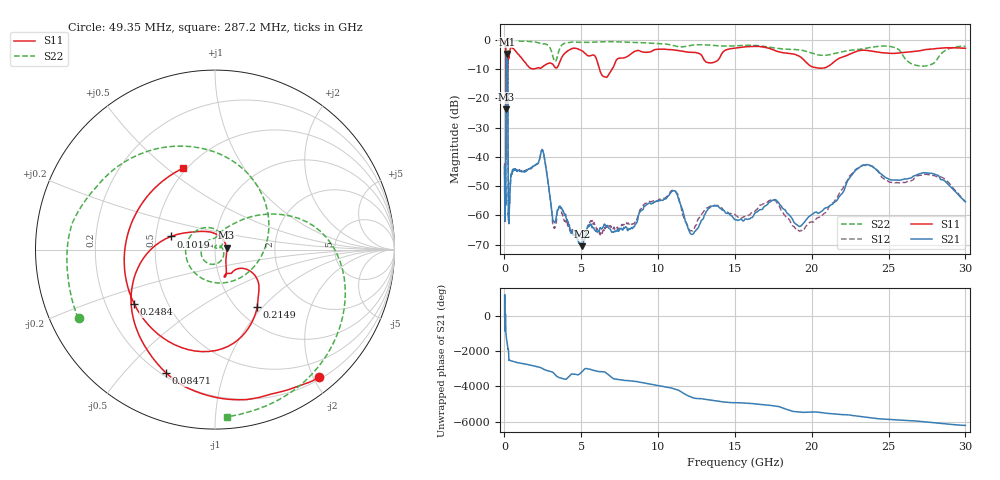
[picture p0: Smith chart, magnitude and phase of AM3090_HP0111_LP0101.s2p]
! Date/Time: Thu, Feb 28, 2019 2:01 PM
! Network Analyzer: Agilent Technologies E8364B Rev: A.07.50.67
! Sweep from 0.010 to 30.000 GHz, 1601 Points, Sweep Type: LOG
! Power Supply: 5.023 V, 0.002 A
# Hz S DB R 50
!freq MagS11 AngS11 MagS21 AngS21 MagS12 AngS12 MagS22 AngS22
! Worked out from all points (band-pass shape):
!   1601 points, 10 MHz to 30 GHz, reference 50 ohm
!   highest |S21| = -4.75 dB at 153.7 MHz (marker M1); lowest = -70.6 dB at 5.077 GHz (marker M2)
!   |S21| within 3 dB of the highest: 113.2 MHz to 202.8 MHz (89.6 MHz wide, 56.7 % of centre)
!   lowest |S11| = -23.7 dB at 109.9 MHz (marker M3), VSWR 1.14, Z = 56.8 + j1.22 ohm
!   |S11| at or under -10 dB: 100.8 MHz to 204 MHz (103.2 MHz wide, 67.7 % of centre); 6.184 GHz to 7.009 GHz (825 MHz wide, 12.5 % of centre)
!   |S22| runs from -40.8 to -0.1 dB; largest |S21 - S12| = 0.013
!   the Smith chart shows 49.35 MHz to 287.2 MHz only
!   S11 on the Smith chart (normalised r, x): 49.35 MHz: 0.23, -2.09; 84.71 MHz: 0.22, -0.66; 101.9 MHz: 0.60, +0.09; 214.9 MHz: 1.23, -0.93; 248.4 MHz: 0.32, -0.27; 287.2 MHz: 0.48, +0.57
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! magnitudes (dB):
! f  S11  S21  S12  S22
! 10 MHz  -0.3  -47.2  -42.2  -0.6
! 38.04 MHz  -0.5  -60.3  -61.3  -1.3
! 49.35 MHz  -0.7  -50.5  -47.1  -1.4
! 84.71 MHz  -2.6  -51.2  -49.8  -5.3
! 101.9 MHz  -11.9  -17.1  -17.1  -15.1
! 109.9 MHz  -23.7  -9.1  -9.1  -16.5
! 133.6 MHz  -15.9  -5.2  -5.2  -40.5
! 144.7 MHz  -16.4  -4.8  -4.8  -29.8
! 153.7 MHz  -16.4  -4.8  -4.7  -24.6
! 214.9 MHz  -8.1  -12.9  -12.9  -11.3
! 248.4 MHz  -5.3  -55.0  -56.1  -1.4
! 287.2 MHz  -6.2  -62.5  -60.4  -0.6
! 550.5 MHz  -2.9  -44.6  -44.5  -0.2
! 2.084 GHz  -9.7  -42.6  -42.5  -0.7
! 2.507 GHz  -9.1  -38.0  -38.0  -1.3
! 5.077 GHz  -3.8  -70.6  -68.0  -0.8
! 7.926 GHz  -5.8  -64.1  -62.6  -0.7
! 10.86 GHz  -3.3  -52.0  -51.6  -1.7
! 12.25 GHz  -4.2  -66.5  -65.4  -1.7
! 19.41 GHz  -6.4  -63.0  -65.4  -3.6
! 23.48 GHz  -3.5  -42.8  -42.9  -2.9
! 30 GHz  -2.8  -55.4  -55.5  -2.1
